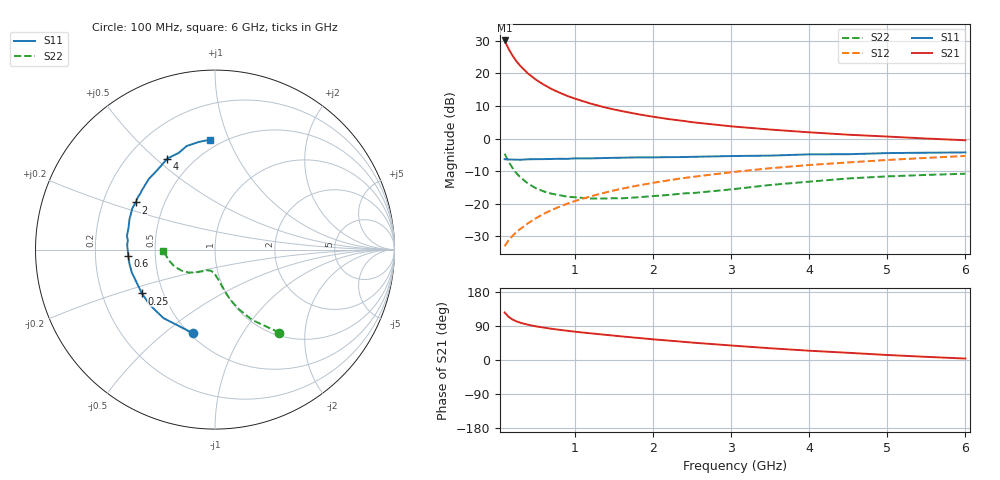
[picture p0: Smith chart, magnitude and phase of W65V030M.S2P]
! SIEMENS Small Signal Semiconductors
! BFR193W
! Si NPN RF Bipolar Junction Transistor in SOT323
! VCE = 5 V  IC = 30 mA
! Common Emitter S-Parameters:  September  1992
# GHz  S  MA  R  50
!  f  S11  S21  S12  S22
! GHz  MAG  ANG  MAG  ANG  MAG  ANG  MAG  ANG
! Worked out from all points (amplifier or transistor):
!   28 points, 100 MHz to 6 GHz, reference 50 ohm
!   highest |S21| = 30.1 dB at 100 MHz (marker M1)
!   |S21| within 3 dB of that: start of sweep to 161.2 MHz
!   unconditionally stable (mu >= 1): 664 MHz to 2.52 GHz
!   at 300 MHz: K = 0.84, MSG = 25.0 dB, |S12| = -27.7 dB
!   at 1.5 GHz: K = 1.03, MAG = 11.3 dB, |S12| = -15.9 dB
!   at 6 GHz: K = 0.91, MSG = 2.4 dB, |S12| = -5.3 dB
!   lowest NFmin = 1.90 dB at 450 MHz
!   S11 on the Smith chart (normalised r, x): 100 MHz: 0.52, -0.63; 250 MHz: 0.38, -0.24; 600 MHz: 0.35, -0.03; 2 GHz: 0.34, +0.24; 4 GHz: 0.36, +0.55; 6 GHz: 0.44, +0.86
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0.1  0.4819 -104.9  31.91 125.4  0.0224 59.1  0.5861 -52.2
0.15  0.4778 -127.1  23.83 114.1  0.0275 58.2  0.4429 -62.2
0.2  0.4761 -140.0  18.78 106.9  0.0321 59.3  0.3554 -68.4
0.25  0.4748 -149.0  15.4 102.1  0.0367 60.7  0.2949 -72.8
0.3  0.4731 -155.2  13.04 98.4  0.041 62.8  0.2564 -75.4
0.4  0.4809 -164.7  9.919 93.0  0.0503 65.3  0.2038 -79.6
0.5  0.4833 -170.6  8.009 88.9  0.06 67.5  0.1733 -82.6
0.6  0.4844 -175.7  6.715 85.5  0.0701 68.6  0.155 -86.2
0.7  0.4861 -179.5  5.758 82.5  0.08 69.3  0.143 -88.4
0.8  0.4901 177.0  5.073 79.7  0.0899 69.8  0.1357 -91.2
0.9  0.4884 173.9  4.517 77.2  0.1 70.0  0.1287 -93.1
1  0.4965 171.1  4.096 74.7  0.1102 70.0  0.1258 -95.3
1.2  0.4967 165.9  3.44 70.4  0.13 69.3  0.1205 -100.7
1.5  0.5064 159.9  2.793 64.3  0.1601 68.1  0.1216 -107.4
2  0.5141 149.3  2.16 54.6  0.2096 65.1  0.1312 -116.3
2.2  0.5193 145.9  1.99 51.2  0.2291 63.7  0.1367 -118.8
3  0.5393 133.2  1.54 38.3  0.3047 57.5  0.1662 -130.1
3.5  0.5476 125.8  1.374 31.0  0.3509 53.3  0.1942 -138.8
4  0.5724 117.7  1.247 24.5  0.3932 48.9  0.2184 -147.2
4.5  0.5753 110.7  1.146 19.0  0.4306 44.7  0.2447 -157.2
5.5  0.6066 98.5  1.001 8.3  0.5052 36.5  0.2773 -174.1
6  0.6128 92.6  0.942 3.8  0.5413 32.2  0.2889 -178.9
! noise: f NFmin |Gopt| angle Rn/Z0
0.45  1.9  0.4  180  0.09
0.9  1.95  0.43  -173  0.11
1.8  2.4  0.58  -144  0.24
